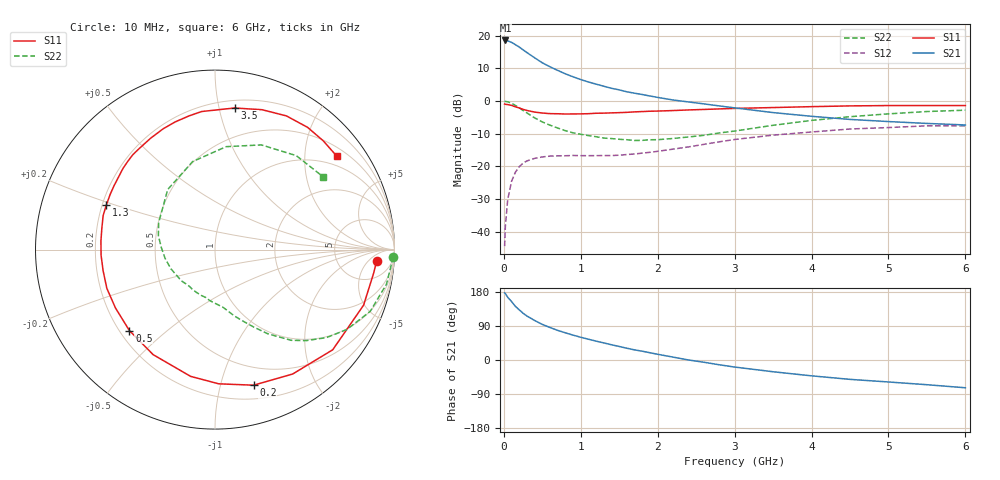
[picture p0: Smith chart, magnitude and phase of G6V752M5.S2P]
! SIEMENS Small Signal Semiconductors
! BFG193
! Si NPN RF Bipolar Junction Transistor in SOT223
! VCE = 0.75 V  IC = 2.5 mA
! Common Emitter S-Parameters:  August  1996
# GHz  S  MA  R  50
!  f  S11  S21  S12  S22
! GHz  MAG  ANG  MAG  ANG  MAG  ANG  MAG  ANG
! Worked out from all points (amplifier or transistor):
!   36 points, 10 MHz to 6 GHz, reference 50 ohm
!   highest |S21| = 18.6 dB at 20 MHz (marker M1)
!   |S21| within 3 dB of that: start of sweep to 257.6 MHz
!   unconditionally stable (mu >= 1): 1.279 GHz to 3.54 GHz; 5.591 GHz to end of sweep
!   at 250 MHz: K = 0.22, MSG = 17.4 dB, |S12| = -19.0 dB
!   at 1.4 GHz: K = 1.08, MAG = 8.6 dB, |S12| = -16.7 dB
!   at 6 GHz: K = 1.01, MAG = -0.5 dB, |S12| = -7.6 dB
!   S11 on the Smith chart (normalised r, x): 10 MHz: 13, -9; 200 MHz: 0.32, -1.27; 500 MHz: 0.24, -0.38; 1.3 GHz: 0.22, +0.19; 3.5 GHz: 0.26, +1.11; 6 GHz: 0.72, +2.79
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0.01  0.9023 -4.2  8.432 177.1  0.006 90.6  0.992 -2.3
0.02  0.8937 -8.4  8.489 175.3  0.0122 85.2  0.987 -4.5
0.05  0.8839 -20.5  8.362 165.7  0.0308 78.7  0.9746 -11.4
0.1  0.8612 -40.4  7.945 154.3  0.059 68.8  0.9308 -21.7
0.15  0.8172 -58.0  7.318 141.6  0.0813 58.1  0.8592 -31.2
0.2  0.7855 -74.1  6.734 132.4  0.0987 50.9  0.7912 -38.3
0.25  0.7481 -88.4  6.098 123.4  0.1122 44.1  0.7183 -44.9
0.3  0.7192 -100.9  5.543 116.1  0.1212 39.0  0.6597 -50.0
0.4  0.6792 -120.5  4.607 104.3  0.1327 31.1  0.5537 -57.9
0.5  0.6564 -136.6  3.861 94.0  0.1396 25.2  0.4795 -63.7
0.6  0.6429 -149.6  3.354 85.7  0.1437 21.3  0.4278 -68.6
0.7  0.6401 -160.3  2.954 78.2  0.145 18.4  0.387 -73.5
0.9  0.6355 -177.1  2.355 65.6  0.147 15.1  0.3268 -81.6
1.1  0.6418 169.1  1.961 54.8  0.146 13.5  0.2961 -91.3
1.3  0.6544 157.6  1.689 45.0  0.1466 13.5  0.2715 -101.0
1.7  0.6839 138.5  1.321 26.7  0.1549 16.4  0.2495 -124.9
2.2  0.7166 120.1  1.04 7.6  0.1838 17.1  0.2676 -156.3
2.8  0.7591 100.9  0.844 -12.6  0.238 12.4  0.3251 166.1
3.5  0.7965 82.1  0.667 -31.0  0.3012 -1.3  0.4261 128.2
4.5  0.8445 61.9  0.524 -51.1  0.3737 -21.5  0.5769 83.8
5.5  0.8549 45.2  0.455 -65.2  0.418 -45.9  0.6923 49.1
6  0.8554 37.4  0.431 -73.3  0.4181 -59.4  0.726 34.0
